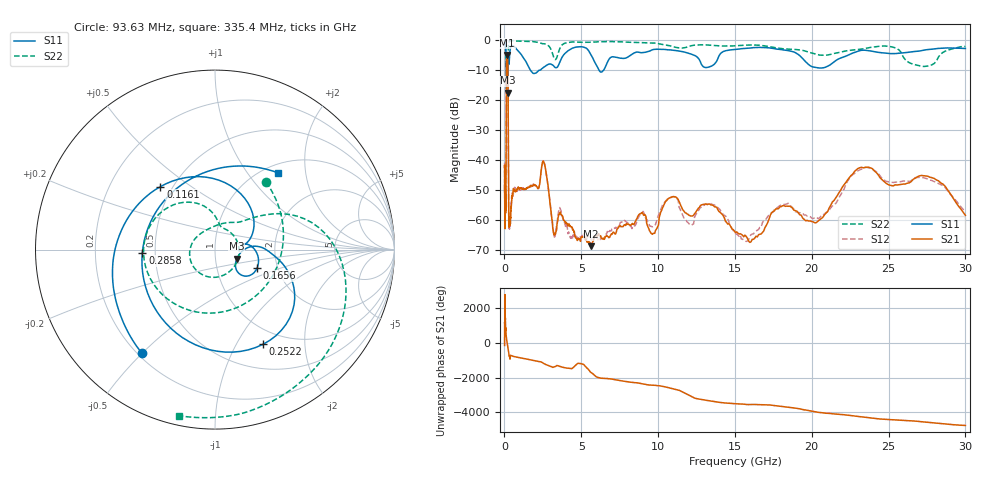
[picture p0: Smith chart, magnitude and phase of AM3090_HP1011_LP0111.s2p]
! Date/Time: Thu, Feb 28, 2019 2:05 PM
! Network Analyzer: Agilent Technologies E8364B Rev: A.07.50.67
! Sweep from 0.010 to 30.000 GHz, 1601 Points, Sweep Type: LOG
! Power Supply: 5.023 V, 0.002 A
# Hz S DB R 50
!freq MagS11 AngS11 MagS21 AngS21 MagS12 AngS12 MagS22 AngS22
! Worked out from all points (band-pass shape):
!   1601 points, 10 MHz to 30 GHz, reference 50 ohm
!   highest |S21| = -5.06 dB at 169.8 MHz (marker M1); lowest = -68.8 dB at 5.64 GHz (marker M2)
!   |S21| within 3 dB of the highest: 131 MHz to 220.6 MHz (89.58 MHz wide, 51 % of centre)
!   lowest |S11| = -17.6 dB at 200.3 MHz (marker M3), VSWR 1.30, Z = 63.4 - j6.59 ohm
!   |S11| at or under -10 dB: 125.2 MHz to 224.3 MHz (99.07 MHz wide, 56.7 % of centre); 1.677 GHz to 2.351 GHz (673.8 MHz wide, 33.4 % of centre); 6.143 GHz to 6.466 GHz (322.3 MHz wide, 5.11 % of centre)
!   |S22| runs from -18.5 to -0.2 dB; largest |S21 - S12| = 0.015
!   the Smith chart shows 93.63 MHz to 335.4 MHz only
!   S11 on the Smith chart (normalised r, x): 93.63 MHz: 0.22, -0.50; 116.1 MHz: 0.43, +0.38; 165.6 MHz: 1.57, -0.34; 252.2 MHz: 0.80, -1.29; 285.8 MHz: 0.42, -0.02; 335.4 MHz: 1.15, +1.42
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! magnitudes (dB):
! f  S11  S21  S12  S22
! 10 MHz  -0.2  -42.4  -41.0  -0.6
! 38.04 MHz  -0.4  -62.2  -59.4  -1.4
! 93.63 MHz  -3.0  -56.3  -54.1  -6.5
! 116.1 MHz  -6.7  -21.1  -21.1  -8.1
! 144.7 MHz  -14.9  -5.7  -5.7  -17.9
! 165.6 MHz  -11.8  -5.1  -5.0  -16.7
! 169.8 MHz  -11.9  -5.1  -5.0  -16.3
! 200.3 MHz  -17.6  -5.7  -5.7  -18.5
! 229.3 MHz  -8.9  -11.2  -11.1  -11.7
! 252.2 MHz  -4.6  -35.0  -35.2  -2.7
! 285.8 MHz  -7.8  -62.0  -60.2  -1.0
! 335.4 MHz  -5.1  -59.0  -62.1  -0.5
! 550.5 MHz  -2.0  -50.9  -52.3  -0.3
! 2.084 GHz  -10.9  -48.8  -49.1  -0.7
! 2.558 GHz  -9.1  -40.7  -40.7  -1.3
! 3.22 GHz  -8.8  -64.5  -64.7  -6.0
! 5.64 GHz  -5.0  -68.8  -66.5  -0.8
! 7.926 GHz  -6.0  -61.4  -60.7  -0.7
! 10.92 GHz  -3.4  -52.3  -52.3  -2.1
! 16.13 GHz  -2.6  -66.5  -64.8  -1.7
! 23.36 GHz  -3.4  -42.7  -42.8  -3.0
! 30 GHz  -2.9  -58.5  -57.4  -2.2
